(* Logix 5000 DataType export ZE2AI_Seneca_OutData; software revision 35.00 *)

TYPE ZE2AI_Seneca_OutData :   // User Define Data Out Type for Seneca ZE-2AI-E Device
STRUCT
   CMD : INT;   // Command Register
   CMD_AUX : UDINT;   // Command Auxiliar
END_STRUCT
END_TYPE
